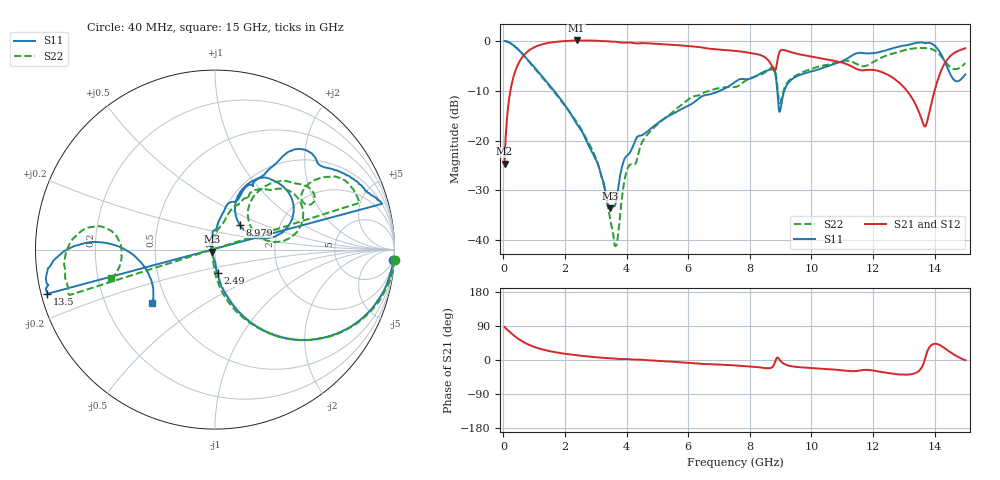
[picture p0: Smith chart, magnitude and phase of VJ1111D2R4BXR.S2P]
! VJ1111D2R4BXR
! DATE 03/08/2022  10:57
! CAPACITORS MOUNTED IN SERIES ON 25 MIL THICK MICROSTRIP SUBSTRATE
# GHz  S  MA  R  50.00
!  FREQ  S11M  S11A  S21M  S21A  S12M  S12A  S22M  S22A
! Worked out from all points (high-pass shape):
!   801 points, 40 MHz to 15 GHz, reference 50 ohm
!   highest |S21| = 0.09 dB at 2.377 GHz (marker M1); lowest = -24.7 dB at 40 MHz (marker M2)
!   |S21| within 3 dB of the highest: 661.6 MHz to 8.376 GHz (7.714 GHz wide, 171 % of centre); 8.93 GHz to 9.798 GHz (868.3 MHz wide, 9.27 % of centre)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
!   lowest |S11| = -33.6 dB at 3.462 GHz (marker M3), VSWR 1.04, Z = 48.3 - j1.17 ohm
!   |S11| at or under -10 dB: 1.644 GHz to 7.038 GHz (5.394 GHz wide, 124 % of centre); 8.893 GHz to 9.122 GHz (229.3 MHz wide, 2.55 % of centre)
!   |S22| runs from -41.2 to 0.0 dB; largest |S21 - S12| = 0.011
!   S11 on the Smith chart (normalised r, x): 40 MHz: 2, -34; 2.49 GHz: 0.99, -0.27; 8.979 GHz: 1.26, +0.36; 13.5 GHz: 0.02, -0.13; 15 GHz: 0.41, -0.31
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0.04  0.9959 -3.4  0.05853 87.5  0.05789 86.0  1.004 -3.2
0.2457  0.9407 -19.3  0.3381 71.0  0.3383 71.2  0.9471 -19.3
0.5823  0.7632 -40.4  0.6643 50.7  0.6631 50.8  0.7622 -40.7
1.3116  0.4214 -66.0  0.933 26.9  0.9309 26.9  0.4116 -67.4
2.3775  0.1477 -83.0  1.011 12.4  1.008 12.5  0.1541 -87.4
2.4897  0.1318 -83.8  1.009 11.3  1.007 11.4  0.1363 -89.7
2.5458  0.1246 -85.3  1.008 10.9  1.005 11.0  0.1264 -90.7
3.0694  0.05813 -94.6  1.002 6.8  0.9986 6.9  0.05814 -102.5
3.4621  0.02083 -144.6  0.9881 4.4  0.9857 4.5  0.01664 -127.8
3.6678  0.02526 146.2  0.9803 3.3  0.9779 3.4  0.00881 128.3
4.0231  0.07109 102.0  0.9631 2.4  0.9612 2.5  0.05171 97.4
5.0329  0.1508 83.4  0.9315 -2.4  0.9287 -2.2  0.1473 74.1
7.52  0.3866 63.9  0.795 -14.3  0.793 -14.1  0.3441 56.9
8.7355  0.5185 37.7  0.5447 -18.5  0.543 -18.2  0.5445 30.6
8.9786  0.1951 45.3  0.7878 -0.3  0.7837 -0.1  0.2363 31.6
10.0258  0.4965 56.9  0.6941 -21.4  0.69 -21.2  0.5272 46.5
12.5129  0.8221 31.9  0.4522 -34.7  0.4504 -34.4  0.725 33.6
13.4105  0.9578 16.4  0.2208 -33.2  0.2199 -32.9  0.8447 20.6
13.504  0.9667 -165.2  0.1892 -27.8  0.1881 -27.3  0.8493 -162.6
13.5788  0.9676 -166.7  0.1634 -20.2  0.1625 -19.7  0.8478 -165.3
14.2707  0.6773 176.4  0.5517 34.3  0.5493 34.8  0.668 168.9
15  0.4607 -139.4  0.8449 -0.7  0.8432 -0.1  0.5989 -164.7
